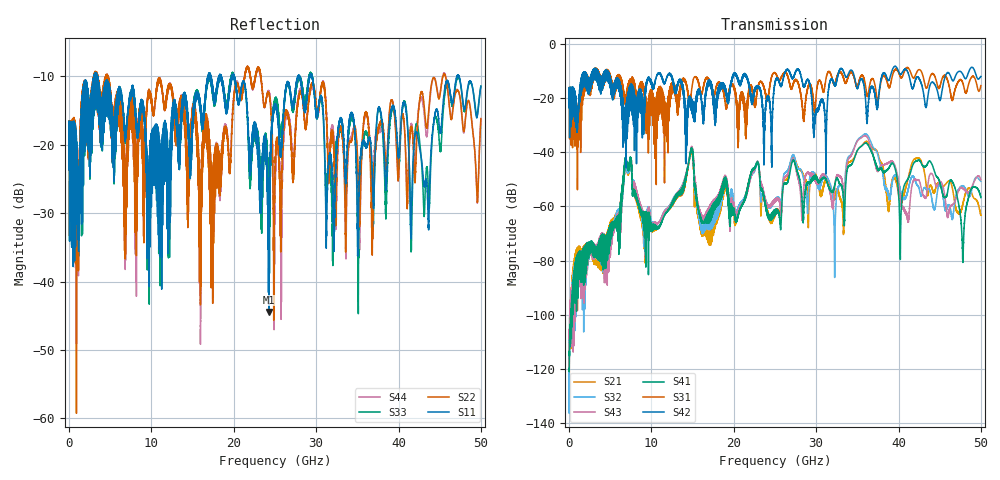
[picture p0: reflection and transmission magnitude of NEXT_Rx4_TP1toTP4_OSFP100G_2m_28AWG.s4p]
! Touchstone data
! Created: 27-Feb-2019 by IdEM 12 (12.1.0)
! COMMENTS
!  Created Wed Feb 27 12:03:36 2019
!  64 Port Network Data from SP1.SP block
!  freq  magS1_1  angS1_1  magS1_2  angS1_2  magS1_3  angS1_3  magS1_4  angS1_4
!  magS1_5  angS1_5  magS1_6  angS1_6  magS1_7  angS1_7  magS1_8  angS1_8
!  magS1_9  angS1_9  magS1_10  angS1_10  magS1_11  angS1_11  magS1_12  angS1_12
!  magS1_13  angS1_13  magS1_14  angS1_14  magS1_15  angS1_15  magS1_16  angS1_16
!  magS1_17  angS1_17  magS1_18  angS1_18  magS1_19  angS1_19  magS1_20  angS1_20
!  magS1_21  angS1_21  magS1_22  angS1_22  magS1_23  angS1_23  magS1_24  angS1_24
!  magS1_25  angS1_25  magS1_26  angS1_26  magS1_27  angS1_27  magS1_28  angS1_28
!  magS1_29  angS1_29  magS1_30  angS1_30  magS1_31  angS1_31  magS1_32  angS1_32
!  magS1_33  angS1_33  magS1_34  angS1_34  magS1_35  angS1_35  magS1_36  angS1_36
!  magS1_37  angS1_37  magS1_38  angS1_38  magS1_39  angS1_39  magS1_40  angS1_40
!  magS1_41  angS1_41  magS1_42  angS1_42  magS1_43  angS1_43  magS1_44  angS1_44
!  magS1_45  angS1_45  magS1_46  angS1_46  magS1_47  angS1_47  magS1_48  angS1_48
!  magS1_49  angS1_49  magS1_50  angS1_50  magS1_51  angS1_51  magS1_52  angS1_52
!  magS1_53  angS1_53  magS1_54  angS1_54  magS1_55  angS1_55  magS1_56  angS1_56
!  magS1_57  angS1_57  magS1_58  angS1_58  magS1_59  angS1_59  magS1_60  angS1_60
!  magS1_61  angS1_61  magS1_62  angS1_62  magS1_63  angS1_63  magS1_64  angS1_64
!  magS2_1  angS2_1  magS2_2  angS2_2  magS2_3  angS2_3  magS2_4  angS2_4
!  magS2_5  angS2_5  magS2_6  angS2_6  magS2_7  angS2_7  magS2_8  angS2_8
!  magS2_9  angS2_9  magS2_10  angS2_10  magS2_11  angS2_11  magS2_12  angS2_12
!  magS2_13  angS2_13  magS2_14  angS2_14  magS2_15  angS2_15  magS2_16  angS2_16
!  magS2_17  angS2_17  magS2_18  angS2_18  magS2_19  angS2_19  magS2_20  angS2_20
!  magS2_21  angS2_21  magS2_22  angS2_22  magS2_23  angS2_23  magS2_24  angS2_24
!  magS2_25  angS2_25  magS2_26  angS2_26  magS2_27  angS2_27  magS2_28  angS2_28
!  magS2_29  angS2_29  magS2_30  angS2_30  magS2_31  angS2_31  magS2_32  angS2_32
!  magS2_33  angS2_33  magS2_34  angS2_34  magS2_35  angS2_35  magS2_36  angS2_36
!  magS2_37  angS2_37  magS2_38  angS2_38  magS2_39  angS2_39  magS2_40  angS2_40
!  magS2_41  angS2_41  magS2_42  angS2_42  magS2_43  angS2_43  magS2_44  angS2_44
!  magS2_45  angS2_45  magS2_46  angS2_46  magS2_47  angS2_47  magS2_48  angS2_48
!  magS2_49  angS2_49  magS2_50  angS2_50  magS2_51  angS2_51  magS2_52  angS2_52
!  magS2_53  angS2_53  magS2_54  angS2_54  magS2_55  angS2_55  magS2_56  angS2_56
!  magS2_57  angS2_57  magS2_58  angS2_58  magS2_59  angS2_59  magS2_60  angS2_60
!  magS2_61  angS2_61  magS2_62  angS2_62  magS2_63  angS2_63  magS2_64  angS2_64
!  magS3_1  angS3_1  magS3_2  angS3_2  magS3_3  angS3_3  magS3_4  angS3_4
!  magS3_5  angS3_5  magS3_6  angS3_6  magS3_7  angS3_7  magS3_8  angS3_8
!  magS3_9  angS3_9  magS3_10  angS3_10  magS3_11  angS3_11  magS3_12  angS3_12
!  magS3_13  angS3_13  magS3_14  angS3_14  magS3_15  angS3_15  magS3_16  angS3_16
!  magS3_17  angS3_17  magS3_18  angS3_18  magS3_19  angS3_19  magS3_20  angS3_20
!  magS3_21  angS3_21  magS3_22  angS3_22  magS3_23  angS3_23  magS3_24  angS3_24
!  magS3_25  angS3_25  magS3_26  angS3_26  magS3_27  angS3_27  magS3_28  angS3_28
!  magS3_29  angS3_29  magS3_30  angS3_30  magS3_31  angS3_31  magS3_32  angS3_32
!  magS3_33  angS3_33  magS3_34  angS3_34  magS3_35  angS3_35  magS3_36  angS3_36
!  magS3_37  angS3_37  magS3_38  angS3_38  magS3_39  angS3_39  magS3_40  angS3_40
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# Hz S MA R 50
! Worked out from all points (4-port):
!   5000 points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, 10 MHz to 50 GHz, reference 50 ohm
!   strongest paths, dB at 10 MHz, 12.51 GHz, 25.01 GHz, 37.51 GHz, 50 GHz:
!     S42: -18.0, -12.6, -14.0, -21.6, -12.0
!     S31: -18.0, -15.9, -10.7, -20.7, -15.4
!     S41: -120.0, -59.5, -63.2, -46.3, -56.7
!     S43: -116.8, -58.9, -58.4, -46.9, -50.2
!     S32: -116.4, -59.2, -57.7, -41.2, -50.7
!     S21: -117.2, -60.0, -63.0, -40.7, -63.3
!   lowest |S11| = -44.4 dB at 24.26 GHz (marker M1), VSWR 1.01, Z = 49.6 - j0.401 ohm
!   |S11| at or under -10 dB: 3.451 GHz to 16.86 GHz (13.4 GHz wide, 132 % of centre); 20.09 GHz to 27.79 GHz (7.695 GHz wide, 32.1 % of centre); 29.5 GHz to 47.1 GHz (17.61 GHz wide, 46 % of centre)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
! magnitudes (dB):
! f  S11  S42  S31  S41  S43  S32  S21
! 10 MHz  -17.7  -18.0  -18.0  -120.0  -116.8  -116.4  -117.2
! 6.97 GHz  -17.6  -25.7  -20.2  -44.0  -43.7  -45.4  -45.8
! 24.26 GHz  -44.4  -20.2  -18.3  -64.9  -60.3  -60.5  -64.4
! 32.26 GHz  -29.2  -15.3  -14.8  -52.0  -52.4  -76.8  -56.6
! 36.08 GHz  -20.1  -24.8  -17.2  -36.6  -34.0  -33.3  -36.0
! 41.04 GHz  -16.5  -9.9  -8.7  -50.3  -63.2  -55.1  -51.2
! 50 GHz  -11.4  -12.0  -15.4  -56.7  -50.2  -50.7  -63.3
